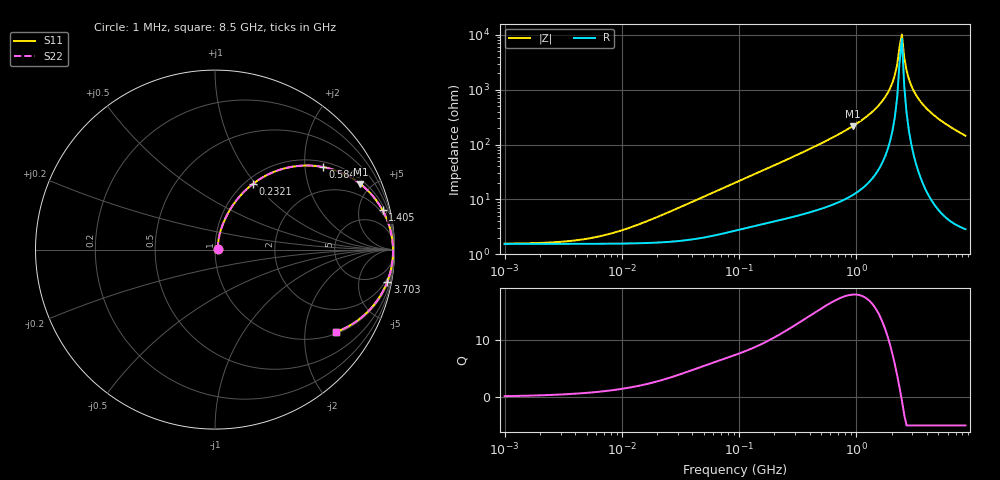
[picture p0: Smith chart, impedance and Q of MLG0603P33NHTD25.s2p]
! S-Parameter Data Generated by TDK Corporation
! Copyright(C) 2025 TDK Corporation.
! All Rights Reserved.
! TDK P/N: MLG0603P33NHTD25 (SMD / SMT Inductor (Coil))
! Property: L=33nH at 300MHz
! Size(LxWxT): 0.6x0.3x0.3mm
! Model Type: s2p (Touchstone File Format Version 1.0)
! Frequency: DC=Yes Start=1MHz Stop=8500MHz 198points Log-sweep
! Model Generated on Feb. 6, 2025
! Terms and conditions regarding TDK Simulation Models:
! 1)This simulation model is being provided solely for informational
!  purposes. Please refer to the specifications of the products in
!  terms of detailed characteristics of such products.
! 2)In no event shall TDK Corporation of any of its subsidiaries be
!  liable for any loss or damage arising, directly or indirectly,
!  from any information contained in this simulation model, including,
!  but not limited to loss or damages arising from any inaccuracies,
!  omissions or errors in connection with such information.
! 3)Any and all copyrights on this simulation model are owned by
!  TDK Corporation.  Duplication or redistribution of this simulation
!  model without prior written permission from TDK Corporation
!  is prohibited.
! 4)This simulation model is subject to any modification or change
!  without any prior notice.
! 5)Neither TDK Corporation nor any of its subsidiaries shall make any
!  warranty, express or implied, including but not limited to the
!  correctness, implied warranties of merchantability and fitness for
!  a particular purpose with respect to this simulation models.
! 6)The use of this simulation model shall be deemed to have consented
!  to the terms and conditions hereof.
! Port Assignments:
!  1 ---@@@--- 2
! Applicable Conditions:
!  Temperature = 25 degC
!  DC Bias Current = 0 A
!  Small Signal Operation
# Hz S MA R 50
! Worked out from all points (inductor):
!   197 points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, 1 MHz to 8.5 GHz, reference 50 ohm
!   read as one part in series: L = 35.6 nH near 23.08 MHz
!   highest Q = 18 at 927.1 MHz (marker M1), where L = 37 nH
!   self-resonance near 2.334 GHz
!   S11 on the Smith chart (normalised r, x): 1 MHz: 1.03, +0.00; 232.1 MHz: 1.09, +0.97; 584.3 MHz: 1.15, +2.48; 1.405 GHz: 1.52, +8.35; 3.703 GHz: 1, -11; 8.5 GHz: 1.06, -2.90
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1000000  0.01543 8.2  0.9847 -0.1  0.9847 -0.1  0.01543 8.2
4587603  0.01839 33.1  0.9846 -0.6  0.9846 -0.6  0.01839 33.1
9168677  0.02554 51.6  0.9843 -1.2  0.9843 -1.2  0.02554 51.6
2.10461e7  0.04921 68.1  0.9827 -2.7  0.9827 -2.7  0.04921 68.1
9.219544e7  0.1919 71.3  0.956 -11.0  0.956 -11.0  0.1919 71.3
2.320976e8  0.4217 60.1  0.8701 -24.8  0.8701 -24.8  0.4217 60.1
4.229561e8  0.6405 46.4  0.7254 -39.7  0.7254 -39.7  0.6405 46.4
5.842944e8  0.7573 37.4  0.6086 -49.1  0.6086 -49.1  0.7573 37.4
9.270694e8  0.8887 24.3  0.4119 -62.5  0.4119 -62.5  0.8887 24.3
1.404574e9  0.9592 13.2  0.2293 -73.2  0.2293 -73.2  0.9592 13.2
1.689417e9  0.9771 8.6  0.1503 -77.0  0.1503 -77.0  0.9771 8.6
1.940355e9  0.9858 5.2  0.09189 -78.5  0.09189 -78.5  0.9858 5.2
2.128028e9  0.9894 3.0  0.05338 -77.1  0.05338 -77.1  0.9894 3.0
2.228565e9  0.9907 1.9  0.03439 -73.3  0.03439 -73.3  0.9907 1.9
2.333852e9  0.9915 0.8  0.01626 -58.0  0.01626 -58.0  0.9915 0.8
2.444114e9  0.9919 -0.3  0.009778 33.6  0.009778 33.6  0.9919 -0.3
2.559585e9  0.9919 -1.4  0.02606 71.1  0.02606 71.1  0.9919 -1.4
2.80715e9  0.9906 -3.7  0.06422 79.8  0.06422 79.8  0.9906 -3.7
3.224109e9  0.9856 -7.1  0.1231 79.8  0.1231 79.8  0.9856 -7.1
3.703002e9  0.9765 -10.5  0.1831 77.4  0.1831 77.4  0.9765 -10.5
5.357206e9  0.9296 -20.5  0.3498 68.3  0.3498 68.3  0.9296 -20.5
8.5e9  0.8159 -34.2  0.5623 54.7  0.5623 54.7  0.8159 -34.2
